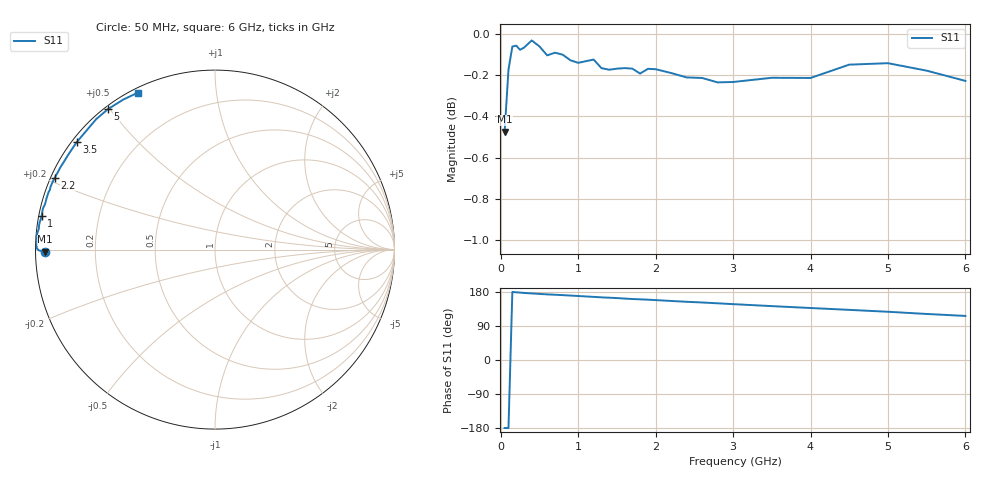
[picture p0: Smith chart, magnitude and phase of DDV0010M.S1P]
! Infineon Technologies  Discrete & RF Semiconductors
! BBY58-02W
! Si Tuning Diode in SCD-80
! VR =
! S-Parameters:  June  2000
# GHz  S  MA  R  50
!  f  S11
! GHz  MAG  ANG
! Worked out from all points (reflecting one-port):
!   34 points, 50 MHz to 6 GHz, reference 50 ohm
!   lowest |S11| = -0.5 dB at 50 MHz (marker M1), VSWR 36.66, Z = 1.36 - j0.305 ohm
!   phase of S11 starts at -179 deg and turns -64 deg over the sweep
!   S11 on the Smith chart (normalised r, x): 50 MHz: 0.03, -0.01; 1 GHz: 0.01, +0.10; 2.2 GHz: 0.01, +0.21; 3.5 GHz: 0.01, +0.34; 5 GHz: 0.01, +0.50; 6 GHz: 0.02, +0.62
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0.05  0.9469 -179.3
0.1  0.9803 -179.7
0.15  0.9931 179.6
0.25  0.9913 177.8
0.3  0.9925 177.0
0.4  0.9965 175.7
0.5  0.9932 174.4
0.6  0.9882 173.2
0.7  0.9897 172.2
0.8  0.9886 171.2
1  0.9841 168.9
1.2  0.9859 166.6
1.3  0.9812 165.3
1.5  0.9809 163.4
1.6  0.9812 162.1
1.7  0.9809 160.9
1.8  0.9782 160.1
1.9  0.9808 159.2
2.2  0.9785 155.8
2.4  0.9761 153.6
2.6  0.9758 151.8
3  0.9736 147.4
3.5  0.9759 142.2
4  0.9758 137.2
4.5  0.9831 132.3
5  0.9839 127.3
5.5  0.9798 121.5
6  0.9742 116.3
